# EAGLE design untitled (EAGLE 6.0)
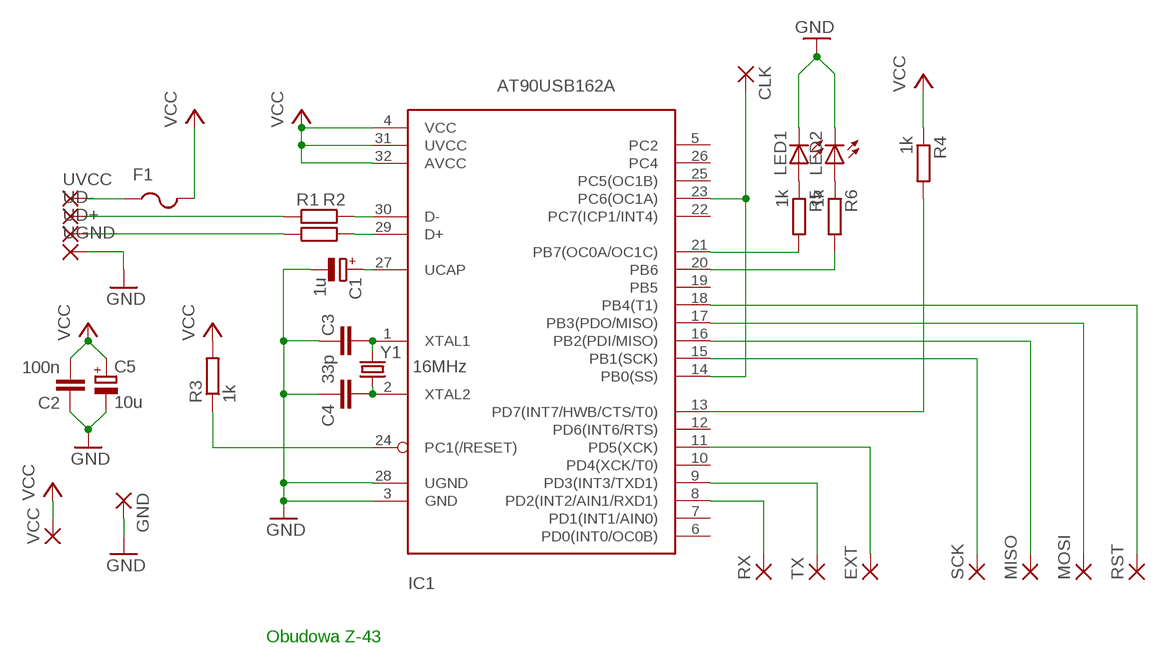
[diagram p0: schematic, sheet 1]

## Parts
C1  1u  CPOL-EUSMCA  [SMC_A]
C2  100n  C-EUC0805  [C0805]
C3  33p  C-EUC1206K  [C1206K]
C4  33p  C-EUC1206K  [C1206K]
C5  10u  CPOL-EUSMCB  [SMC_B]
CLK  SMD2  [SMD1,27-2,54]
EXT  SMD2  [SMD1,27-2,54]
F1  PTCFUSE-1206  [R1206]
GND  SMD2  [SMD1,27-2,54]
IC1  AT90USB162A  [TQFP32-08]
LED1  LEDCHIPLED_1206  [CHIPLED_1206]
LED2  LEDCHIPLED_1206  [CHIPLED_1206]
MISO  SMD2  [SMD1,27-2,54]
MOSI  SMD2  [SMD1,27-2,54]
R1  22  R-EU_M1206  [M1206]
R2  22  R-EU_M1206  [M1206]
R3  1k  R-EU_M1206  [M1206]
R4  1k  R-EU_M1206  [M1206]
R5  1k  R-EU_M1206  [M1206]
R6  1k  R-EU_M1206  [M1206]
RST  SMD2  [SMD1,27-2,54]
RX  SMD2  [SMD1,27-2,54]
SCK  SMD2  [SMD1,27-2,54]
TX  SMD2  [SMD1,27-2,54]
UD+  SMD2  [SMD1,27-2,54]
UD-  SMD2  [SMD1,27-2,54]
UGND  SMD2  [SMD1,27-2,54]
UVCC  SMD2  [SMD1,27-2,54]
VCC  SMD2  [SMD1,27-2,54]
Y1  16MHz  CRYSTAL10.5X4.8  [CRYSTAL-SMD-10.5X4.8-2PIN]

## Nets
DM: IC1.30(D-) R2.2
DP: IC1.29(D+) R1.2
GND: C1.- C2.1 C3.2 C4.2 C5.- GND.1(P) IC1.3(GND) IC1.28(UGND) LED1.C LED2.C UGND.1(P)
N$1: IC1.24(PC1(/RESET)) R3.1
N$2: IC1.13(PD7(INT7/HWB/CTS/T0)) R4.2
N$3: C1.+ IC1.27(UCAP)
N$4: LED1.A R5.1
N$5: LED2.A R6.1
N$6: CLK.1(P) IC1.14(PB0(SS)) IC1.23(PC6(OC1A))
N$7: R1.1 UD+.1(P)
N$8: R2.1 UD-.1(P)
N$9: F1.1 UVCC.1(P)
N$10: IC1.20(PB6) R6.2
N$12: IC1.17(PB3(PDO/MISO)) MOSI.1(P)
N$13: IC1.16(PB2(PDI/MISO)) MISO.1(P)
N$14: IC1.15(PB1(SCK)) SCK.1(P)
N$19: IC1.21(PB7(OC0A/OC1C)) R5.2
N$20: IC1.9(PD3(INT3/TXD1)) TX.1(P)
N$21: IC1.8(PD2(INT2/AIN1/RXD1)) RX.1(P)
N$24: EXT.1(P) IC1.11(PD5(XCK))
N$25: C3.1 IC1.1(XTAL1) Y1.P$2
N$26: C4.1 IC1.2(XTAL2) Y1.P$1
RST: IC1.18(PB4(T1)) RST.1(P)
VCC: C2.2 C5.+ F1.2 IC1.4(VCC) IC1.31(UVCC) IC1.32(AVCC) R3.2 R4.1 VCC.1(P)
Unconnected: IC1.5(PC2) IC1.6(PD0(INT0/OC0B)) IC1.7(PD1(INT1/AIN0)) IC1.10(PD4(XCK/T0)) IC1.12(PD6(INT6/RTS)) IC1.19(PB5) IC1.22(PC7(ICP1/INT4)) IC1.25(PC5(OC1B)) IC1.26(PC4)

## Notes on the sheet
- Obudowa Z-43

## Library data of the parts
C1 C5 = rcl:CPOL-EU: POLARIZED CAPACITOR, European symbol
C2-C4 = rcl:C-EU: CAPACITOR, European symbol
CLK EXT GND MISO MOSI RST RX SCK TX UD+ UD- UGND UVCC VCC = wirepad:SMD2: SMD PAD
F1 = adafruit:PTCFUSE: PTC fuses, resettable thermistors
IC1 = adafruit:AT90USB162: MICROCONTROLLER 8 Kbytes FLASH 1 kbytes SRAM 512 bytes EEPROM USART 6-channel 10 bit ADC 2-channel 8 bit ADC
LED1 LED2 = led:LED: LED
R1-R6 = rcl:R-EU_: RESISTOR, European symbol
Y1 = SparkFun:CRYSTAL: Crystals

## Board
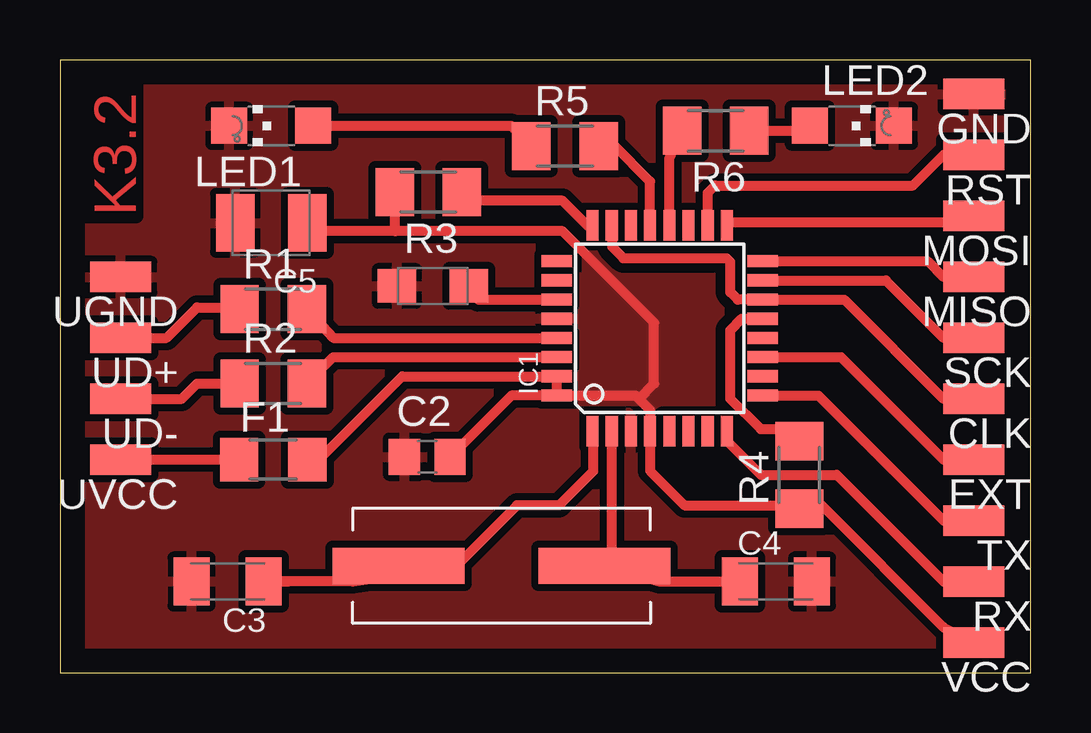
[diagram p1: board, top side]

Size 40.48 x 25.55 mm. Coordinates in mm from the lower left corner, seen from the top.
Outline: 0,0 40.48,0 40.48,25.55 0,25.55 0,0
Copper layers (1*16): Top 0.035mm / dielectric 1.5mm / Bottom 0.035mm
Design rules: minimum track width 10mil, minimum drill 24mil, track to track 8mil, track to pad 8mil, pad to pad 8mil, via to via 8mil, smd to smd 8mil, copper to edge 40mil, drill to drill 8mil, minimum pad ring 10mil, minimum via ring 8mil, stop-mask expansion 4mil, vias tented up to drill 0mil, thermal gap 10mil

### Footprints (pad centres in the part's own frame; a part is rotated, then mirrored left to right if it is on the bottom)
SMC_A = smd 1.6 x 1.4: + -1.5,0; - 1.5,0
C0805 = smd 1.3 x 1.5: 1 -0.95,0; 2 0.95,0
C1206K = smd 1.5 x 2: 1 -1.5,0; 2 1.5,0
SMC_B = smd 1.6 x 2.4: + -1.5,0; - 1.5,0
SMD1,27-2,54 = smd 1.27 x 2.54: 1 0,0
R1206 = smd 1.6 x 1.803: 1 -1.422,0; 2 1.422,0
TQFP32-08 = smd 1.27 x 0.508: 1 -4.293,2.8; 2 -4.293,2; 3 -4.293,1.2; 4 -4.293,0.4; 5 -4.293,-0.4; 6 -4.293,-1.2; 7 -4.293,-2; 8 -4.293,-2.8; 17 4.293,-2.8; 18 4.293,-2; 19 4.293,-1.2; 20 4.293,-0.4; 21 4.293,0.4; 22 4.293,1.2; 23 4.293,2; 24 4.293,2.8 | smd 0.508 x 1.27: 9 -2.8,-4.293; 10 -2,-4.293; 11 -1.2,-4.293; 12 -0.4,-4.293; 13 0.4,-4.293; 14 1.2,-4.293; 15 2,-4.293; 16 2.8,-4.293; 25 2.8,4.293; 26 2,4.293; 27 1.2,4.293; 28 0.4,4.293; 29 -0.4,4.293; 30 -1.2,4.293; 31 -2,4.293; 32 -2.8,4.293
CHIPLED_1206 = smd 1.5 x 1.5: A 0,-1.75; C 0,1.75
M1206 = smd 1.6 x 2: 1 -1.4,0; 2 1.4,0
CRYSTAL-SMD-10.5X4.8-2PIN = smd 5.5 x 1.5: P$1 -4.3,0; P$2 4.3,0

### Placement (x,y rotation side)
C1  15.55,16.13 180 top
C2  15.31,9.01 0 top
C3  6.99,3.81 180 top
C4  29.84,3.81 0 top
C5  8.81,18.76 180 top
CLK  38.1,11.43 90 top
EXT  38.1,8.89 90 top
F1  8.89,8.89 0 top
GND  38.1,24.13 90 top
IC1  25,14.37 90 top
LED1  8.81,22.81 90 top
LED2  33.02,22.81 270 top
MISO  38.1,16.51 90 top
MOSI  38.1,19.05 90 top
R1  8.89,15.16 0 top
R2  8.89,12.06 0 top
R3  15.35,20.04 180 top
R4  30.81,8.26 90 top
R5  21.05,21.97 0 top
R6  27.33,22.6 180 top
RST  38.1,21.59 90 top
RX  38.1,3.81 90 top
SCK  38.1,13.97 90 top
TX  38.1,6.35 90 top
UD+  2.54,13.97 90 top
UD-  2.54,11.43 90 top
UGND  2.54,16.51 90 top
UVCC  2.54,8.89 90 top
VCC  38.1,1.27 90 top
Y1  18.41,4.46 180 top

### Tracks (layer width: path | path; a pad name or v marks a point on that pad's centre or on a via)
DM
  Top 0.406: IC1.30 11.39,13.16 R2.2
DP
  Top 0.406: IC1.29 11.39,13.96 R1.2
GND
  pour Top (isolate 0.305): 0,0 40.01,0 40.01,25.4 0,25.4
N$1
  Top 0.406: IC1.24 21.98,18.66 20.95,19.68 17.03,19.68 R3.1
N$2
  Top 0.406: IC1.13 28.41,14.77 27.94,14.29 27.94,11.43 29.21,10.16 31.11,10.16 30.98,9.65 R4.2
N$3
  Top 0.406: IC1.27 17.45,15.56 17.05,15.97 C1.+
N$4
  Top 0.406: LED1.A 18.81,22.81 R5.1
N$5
  Top 0.406: R6.1 31.06,22.6 LED2.A
N$6
  Top 0.406: IC1.23 23.01,17.77 23.48,17.29 27.79,17.29 27.94,17.13 27.94,15.88 28.25,15.56 IC1.14 32.7,15.56 36.83,11.43 CLK.1
N$7
  Top 0.406: UD+.1 4.45,13.97 5.71,15.24 7.57,15.24 | 7.62,15.24 7.57,15.24 | 7.57,15.24 R1.1
N$8
  Top 0.406: 7.98,12.34 7.62,11.71 7.49,12.21 R2.1 | UD-.1 5.08,11.43 5.71,12.06 R2.1 | R2.1 7.62,12.06
N$9
  Top 0.406: UVCC.1 F1.1
  Top 0.61: 7.19,9.17 F1.1
N$10
  Top 0.406: IC1.20 25.4,21.43 R6.2
N$12
  Top 0.406: IC1.17 27.94,18.8 37.85,18.8 MOSI.1
N$13
  Top 0.406: IC1.16 36.17,17.16 36.83,16.51 MISO.1
N$14
  Top 0.406: IC1.15 34.44,16.36 36.83,13.97 SCK.1
N$19
  Top 0.406: IC1.21 24.6,20.48 23.09,22 R5.2
N$20
  Top 0.406: IC1.9 31.61,11.56 36.83,6.35 TX.1
N$21
  Top 0.406: IC1.8 27.8,9.66 29.21,8.26 32.38,8.26 36.83,3.81 RX.1
N$24
  Top 0.406: IC1.11 32.55,13.16 36.83,8.89 EXT.1
N$25
  Top 0.406: IC1.1 22.23,10.05 22.23,8.4 20.8,6.99 19.05,6.99 16.51,4.45 12.21,3.81 | 12.21,3.81 C3.1 9.53,3.81 | Y1.P$2 12.21,3.81
N$26
  Top 0.406: IC1.2 23,4.45 23.64,4.24 Y1.P$1 25,3.81 C4.1
RST
  Top 0.406: IC1.18 27,20.02 27.3,20.32 35.56,20.32 36.83,21.59 RST.1
VCC
  Top 0.406: IC1.32 IC1.31 14.27,12.37 10.95,9.04 F1.2 | IC1.32 24,11.56 24.13,11.43 | 24.13,11.43 24.6,10.96 IC1.4 24.6,8.42 26.04,6.99 31.58,6.99 | 13.97,18.41 20.95,18.41 24.77,14.61 24.77,12.06 24.13,11.43 | 31.58,6.99 31.75,6.99 36.83,1.91 VCC.1 | 31.58,6.99 R4.1 | IC1.32 18.81,11.56 C2.2 | C5.+ 10.45,18.76 10.79,18.41 13.97,18.41 | R3.2 13.95,18.43 13.97,18.41
  pour Top (isolate 0.406): 21.59,17.78 21.59,10.79 28.57,10.79 28.57,17.78

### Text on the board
Top: K3.2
